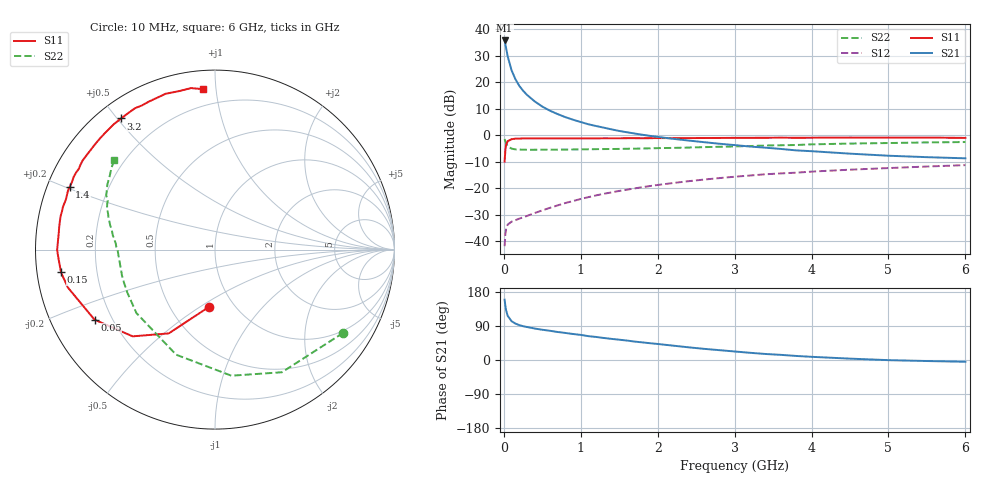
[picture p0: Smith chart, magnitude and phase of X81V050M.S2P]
! SIEMENS Small Signal Semiconductors
! BFP136W
! Si NPN RF Bipolar Junction Transistor in SOT343
! VCE = 1 V  IC = 50 mA
! Common Emitter S-Parameters:  September  1994
# GHz  S  MA  R  50
!  f  S11  S21  S12  S22
! GHz  MAG  ANG  MAG  ANG  MAG  ANG  MAG  ANG
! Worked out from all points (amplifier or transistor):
!   40 points, 10 MHz to 6 GHz, reference 50 ohm
!   highest |S21| = 35.8 dB at 10 MHz (marker M1)
!   |S21| within 3 dB of that: start of sweep to 30.22 MHz
!   unconditionally stable (mu >= 1): 554.3 MHz to 3.237 GHz; 3.792 GHz to 3.811 GHz; 5.904 GHz to end of sweep
!   at 200 MHz: K = 0.57, MSG = 25.1 dB, |S12| = -31.4 dB
!   at 1.5 GHz: K = 1.14, MAG = 9.0 dB, |S12| = -21.0 dB
!   at 6 GHz: K = 1.01, MAG = 0.7 dB, |S12| = -11.2 dB
!   S11 on the Smith chart (normalised r, x): 10 MHz: 0.77, -0.55; 50 MHz: 0.13, -0.27; 150 MHz: 0.07, -0.07; 1.4 GHz: 0.07, +0.21; 3.2 GHz: 0.07, +0.51; 6 GHz: 0.10, +0.92
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0.01  0.3193 -95.6  61.97 159.2  0.0081 68.9  0.8516 -33.0
0.02  0.5333 -118.9  52.62 142.5  0.0137 55.7  0.7784 -61.4
0.03  0.6663 -133.5  44.03 130.6  0.0175 45.6  0.7084 -82.6
0.05  0.7765 -149.8  31.04 116.6  0.0207 34.8  0.6243 -110.3
0.1  0.8469 -165.6  17.01 102.4  0.0235 28.8  0.5626 -141.1
0.15  0.8672 -171.6  11.55 96.1  0.025 31.0  0.5442 -153.6
0.2  0.8708 -175.2  8.651 92.2  0.0268 32.8  0.5394 -160.3
0.25  0.8754 -177.9  6.979 89.2  0.0284 35.8  0.5381 -164.5
0.3  0.8795 -179.9  5.831 87.1  0.0301 39.0  0.5354 -167.4
0.4  0.876 176.7  4.395 83.1  0.0342 43.7  0.5355 -171.2
0.5  0.8754 173.8  3.499 79.8  0.0384 47.4  0.5363 -173.7
0.6  0.8769 172.1  2.921 77.1  0.0429 50.2  0.5374 -175.4
0.7  0.8787 169.5  2.522 73.9  0.0477 53.0  0.5389 -176.6
0.9  0.8788 166.0  1.976 68.6  0.0576 55.2  0.5416 -179.1
1.1  0.8764 161.6  1.62 62.9  0.0683 56.7  0.5464 179.3
1.4  0.8815 156.7  1.299 55.7  0.084 57.0  0.553 176.9
1.8  0.882 149.3  1.028 46.5  0.1052 55.6  0.5647 173.7
2.2  0.8876 142.7  0.861 37.9  0.1261 53.1  0.5803 170.5
3.2  0.8985 125.6  0.616 19.0  0.1747 44.2  0.6297 161.2
4.5  0.9107 107.6  0.452 3.6  0.2252 32.0  0.701 148.8
5.5  0.9097 98.4  0.388 -2.7  0.2583 24.0  0.7361 141.5
6  0.8959 94.2  0.369 -4.7  0.2746 19.6  0.7491 138.4
